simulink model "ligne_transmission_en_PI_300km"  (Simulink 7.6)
settings: Solver=ode23tb  StartTime=0.0  StopTime=0.2  RelTol=1e-4
PreLoadFcn:
  | clc
  | close all
  | delete *.mat
InitFcn:
  | clc
  | clear all
  | T=1/60;
StopFcn:
  | close all
  | load sortie_ligne.mat
  | plot(x(1,:),x(2,:),x(1,:),x(3,:))
  | grid
  | title('Tension d''entrée et tension en bout de ligne')
  | xlabel('temps')
  | delete *.mat
libraries: powerlib x8, powerlib_extras x1

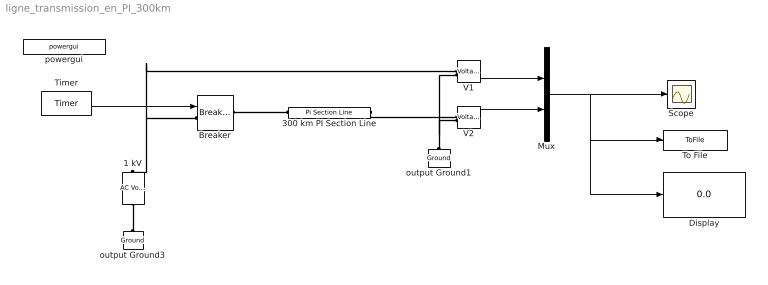
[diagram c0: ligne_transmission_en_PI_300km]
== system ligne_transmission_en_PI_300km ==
  1 kV : powerlib/Electrical Sources/AC Voltage Source  Description=source block  DialogController=POWERSYS.PowerSysDialog  SystemSampleTime=-1  Amplitude=1e3  Phase=0  Frequency=60  SampleTime=0  Measurements=None
  300 km PI Section Line : powerlib/Elements/Pi Section Line  DialogController=POWERSYS.PowerSysDialog  PhysicalDomain=powersysdomain  SubClassName=unknown  LeftPortType=p1  RightPortType=p1  LConnTagsString=__new0  RConnTagsString=__new0  Frequency=60  Resistance=0.0955  Inductance=2.137e-03  Capacitance=12.37e-09  Length=300  PiSections=10  Measurements=None
  Breaker : powerlib/Elements/Breaker  DialogController=POWERSYS.PowerSysDialog  SystemSampleTime=-1  BreakerResistance=0.01  InitialState=1  SnubberResistance=inf  SnubberCapacitance=0  External=on  Measurements=None  MoreParameters=off  NoBreakLoop=off
  Display : Display
  Mux : Mux  Inputs=2
  Scope : Scope
  Timer : powerlib_extras/Control  Blocks/Timer  DialogController=POWERSYS.PowerSysDialog  SystemSampleTime=-1  t="[2*T  3*T ]"  e=[0 1]
  To File : ToFile  Filename=sortie_ligne  MatrixName=x
  V1 : powerlib/Measurements/Voltage Measurement  Tag=PoWeRsYsTeMmEaSuReMeNt  DialogController=POWERSYS.PowerSysDialog  SystemSampleTime=-1  PhasorSimulation=off  OutputType=Magnitude  PSBequivalent=0
  V2 : powerlib/Measurements/Voltage Measurement  Tag=PoWeRsYsTeMmEaSuReMeNt  DialogController=POWERSYS.PowerSysDialog  SystemSampleTime=-1  PhasorSimulation=off  OutputType=Magnitude  PSBequivalent=0
  output Ground1 : powerlib/Elements/Ground  DialogController=POWERSYS.PowerSysDialog  PhysicalDomain=powersysdomain  SubClassName=unknown  LeftPortType=p1  RightPortType=p1  LConnTagsString=a
  output Ground3 : powerlib/Elements/Ground  DialogController=POWERSYS.PowerSysDialog  PhysicalDomain=powersysdomain  SubClassName=unknown  LeftPortType=p1  RightPortType=p1  LConnTagsString=a
  powergui : powerlib/powergui  Priority=2  SystemSampleTime=-1  SimulationMode=Continuous  SampleTime=0  frequency=60  SPID=off  DisableSnubberDevices=off  DisableRonSwitches=off  DisableVfSwitches=off  SwTol=0  Interpol=off  frequencyindice=60  echomessages=off  HookPort=off  DisplayEquations=off  FunctionMessages=off  EnableUseOfTLC=off  x0status=blocks  RestoreLinks=warning  ResistiveCurrentMeasurement=off  Frange=0:2:2000  Ylog=on  Xlog=off  ShowGrid=off  save=off  variable=ZData  ZoomFFT=on  StartTime=0.0  cycles=1  DisplayStyle=off  fundamental=60  FreqAxis=off  MaxFrequency=1000  frequencyindicesteady=1  RmsSteady=1  display=on  Ts=0  methode=off
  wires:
  V2/1 -> Mux/2
  V1/1 -> Mux/1
  Mux/1 -> Scope/1, To File/1, Display/1
  Timer/1 -> Breaker/1
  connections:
  output Ground3/LConn1 -- 1 kV/LConn1
  Breaker/LConn1 -- 1 kV/RConn1 -- V1/LConn1
  Breaker/RConn1 -- 300 km PI Section Line/LConn1
  output Ground1/LConn1 -- V2/LConn2 -- V1/LConn2
  300 km PI Section Line/RConn1 -- V2/LConn1
